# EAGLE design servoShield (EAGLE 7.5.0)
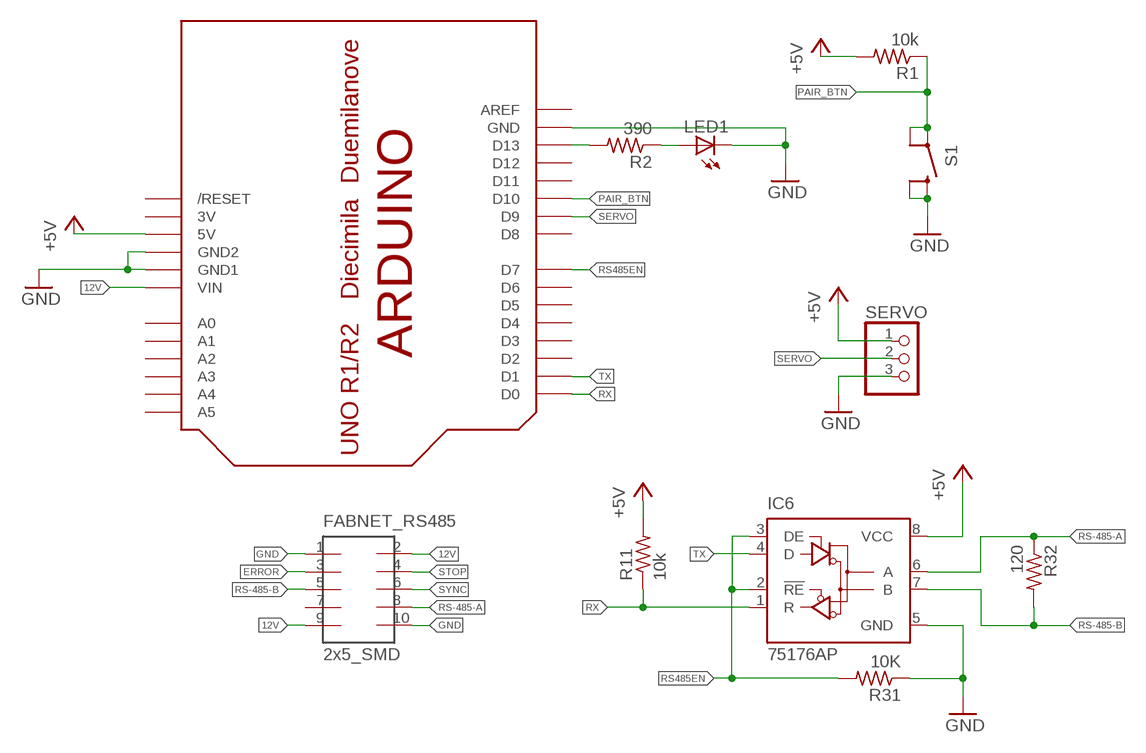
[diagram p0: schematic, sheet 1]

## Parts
FABNET_RS485  2x5_SMD  2X5HEADER  [2X5_SMD]
IC6  75176AP  [DIL08]
LED1  LEDCHIPLED_1206  [CHIPLED_1206]
R1  10k  R-US_R1206  [R1206]
R2  390  R-US_R1206  [R1206]
R11  10k  R-US_R1206  [R1206]
R31  10K  R-US_R1206  [R1206]
R32  120  R-US_R0805  [R0805]
S1  SWITCH-MOMENTARY-2  [TACTILE_SWITCH_TALL]
SERVO  PINHD-1X3  [1X03]
U$1  ARDUINOUNO  [ARDUINO]

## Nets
12V: FABNET_RS485.2 FABNET_RS485.9 U$1.VIN
+5V: IC6.8(VCC) R1.2 R11.2 SERVO.1 U$1.5V
ERROR: FABNET_RS485.3
GND: FABNET_RS485.1 FABNET_RS485.10 IC6.5(GND) LED1.C R31.1 S1.B1 S1.B2 SERVO.3 U$1.GND U$1.GND1 U$1.GND2
N$1: R2.2 U$1.D13
N$2: LED1.A R2.1
PAIR_BTN: R1.1 S1.A1 S1.A2 U$1.D10
RS485EN: IC6.2(!RE) IC6.3(DE) R31.2 U$1.D7
RS-485-A: FABNET_RS485.8 IC6.6(A) R32.1
RS-485-B: FABNET_RS485.5 IC6.7(B) R32.2
RX: IC6.1(R) R11.1 U$1.D0
SERVO: SERVO.2 U$1.D9
STOP: FABNET_RS485.4
SYNC: FABNET_RS485.6
TX: IC6.4(D) U$1.D1
Unconnected: FABNET_RS485.7 U$1.A0 U$1.A1 U$1.A2 U$1.A3 U$1.A4 U$1.A5 U$1.AREF U$1.D2 U$1.D3 U$1.D4 U$1.D5 U$1.D6 U$1.D8 U$1.D11 U$1.D12 U$1.RESET(/RESET)

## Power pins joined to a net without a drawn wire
3V: U$1.3V

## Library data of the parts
FABNET_RS485 = mellis:2X5HEADER
IC6 = 751xx:75176A: DIFFERENTIAL BUS TRANSCEIVER Source: http://focus.ti.com/lit/ds/symlink/sn75176a.pdf
LED1 = led:LED: LED
R1 R2 R11 R31 R32 = rcl:R-US_: RESISTOR, American symbol
S1 = SparkFun-Electromechanical_2:SWITCH-MOMENTARY-2: Various NO switches- pushbuttons, reed, etc
SERVO = pinhead:PINHD-1X3: PIN HEADER
U$1 = adafruit:ARDUINO: Arduino Diecimila/Duemilanove Make a shield with ease, this package has all the named pins as well as the two mounting drill holes and an outline of the USB and DC power connector. The outline is on the DIMENSION layer, so if your board house uses it they will cut the outline to match.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

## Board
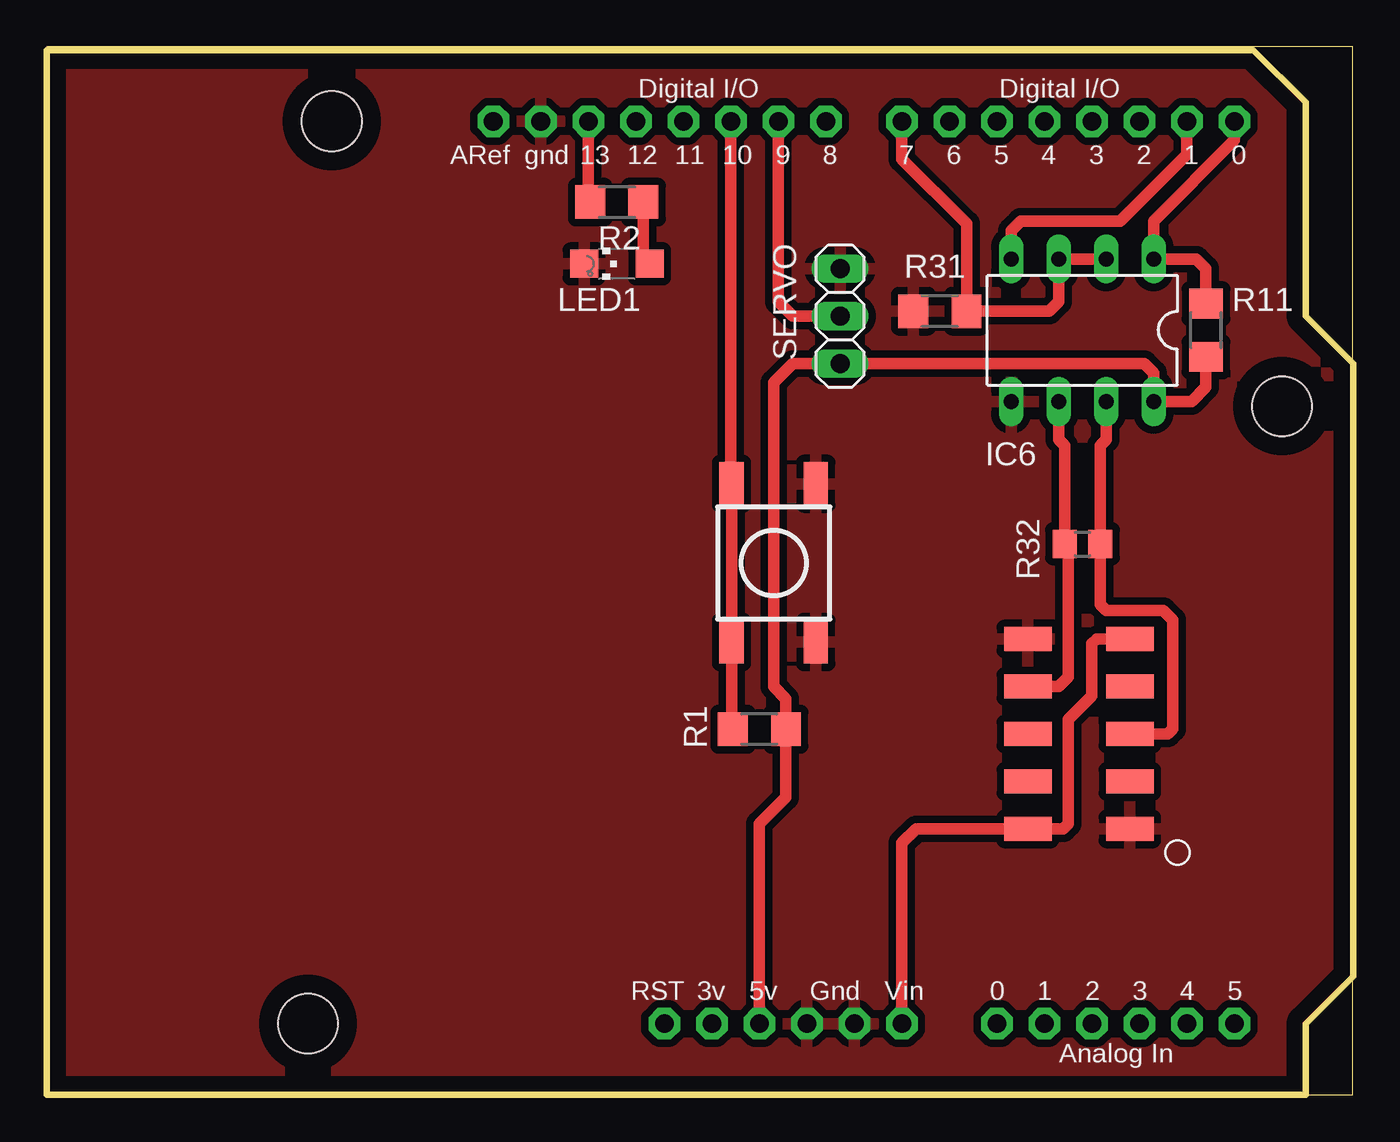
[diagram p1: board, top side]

Size 69.85 x 56.06 mm. Coordinates in mm from the lower left corner, seen from the top.
Outline: 0,0 69.83,0 69.83,56.06 0,56.06 0,0
Copper layers (1*16): Top 0.035mm / dielectric 1.5mm / Bottom 0.035mm
Design rules "default *": minimum track width 10mil, minimum drill 24mil, track to track 16mil, track to pad 16mil, pad to pad 16mil, via to via 16mil, smd to smd 16mil, copper to edge 40mil, drill to drill 8mil, minimum pad ring 10mil, minimum via ring 8mil, stop-mask expansion 4mil, vias tented up to drill 0mil, thermal gap 16mil
Milling: 9 lines

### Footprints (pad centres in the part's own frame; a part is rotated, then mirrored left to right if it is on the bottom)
2X5_SMD = smd 2.54 x 1.27: 1 -2.54,5.08; 2 2.92,5.08; 3 -2.54,2.54; 4 2.92,2.54; 5 -2.54,0; 6 2.92,0; 7 -2.54,-2.54; 8 2.92,-2.54; 9 -2.54,-5.08; 10 2.92,-5.08
DIL08 = drill 0.813 long: 1 -3.81,-3.81; 2 -1.27,-3.81; 3 1.27,-3.81; 4 3.81,-3.81; 5 3.81,3.81; 6 1.27,3.81; 7 -1.27,3.81; 8 -3.81,3.81
CHIPLED_1206 = smd 1.5 x 1.5: A 0,-1.75; C 0,1.75
R1206 = smd 1.6 x 1.803: 1 -1.422,0; 2 1.422,0
R0805 = smd 1.3 x 1.5: 1 -0.95,0; 2 0.95,0
TACTILE_SWITCH_TALL = smd 2.312 x 1.3: A1 -4.229,-2.25; A2 4.229,-2.25; B1 -4.229,2.25; B2 4.229,2.25
1X03 = drill 1.016 long: 1 -2.54,0; 2 0,0; 3 2.54,0
ARDUINO = drill 1 pad 1.676 octagon: 3V 35.56,2.54; 5V 38.1,2.54; A0 50.8,2.54; A1 53.34,2.54; A2 55.88,2.54; A3 58.42,2.54; A4 60.96,2.54; A5 63.5,2.54; AREF 23.876,50.8; D0 63.5,50.8; D1 60.96,50.8; D2 58.42,50.8; D3 55.88,50.8; D4 53.34,50.8; D5 50.8,50.8; D6 48.26,50.8; D7 45.72,50.8; D8 41.656,50.8; D9 39.116,50.8; D10 36.576,50.8; D11 34.036,50.8; D12 31.496,50.8; D13 28.956,50.8; GND 26.416,50.8; GND1 43.18,2.54; GND2 40.64,2.54; RESET 33.02,2.54; VIN 45.72,2.54 | hole 3.2: 15.24,50.8; 66.04,35.56; 13.97,2.54

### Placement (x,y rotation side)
FABNET_RS485  55.37,19.3 180 top
IC6  55.37,40.89 180 top
LED1  30.48,44.45 90 top
R1  38.1,19.56 0 top
R2  30.48,47.75 180 top
R11  61.98,40.89 270 top
R31  47.75,41.91 0 top
R32  55.37,29.46 0 top
S1  38.86,28.45 270 top
SERVO  42.42,41.66 90 top
U$1  0,1.27 0 top

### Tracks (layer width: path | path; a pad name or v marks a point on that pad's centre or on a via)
12V
  Top 0.61: FABNET_RS485.9 56.13,24.38 55.88,24.13 55.88,21.34 54.61,20.07 54.61,14.48 54.36,14.22 FABNET_RS485.2 46.48,14.22 45.72,13.46 U$1.VIN
+5V
  Top 0.61: U$1.5V 38.1,14.48 39.52,15.9 R1.2 39.52,21.18 38.86,21.84 38.86,38.1 39.88,39.12 SERVO.1 58.67,39.12 59.18,38.61 IC6.8 61.21,37.08 61.98,37.85 R11.2
GND
  pour Top: 0,0 67.31,0 67.31,3.81 69.85,6.35 69.85,39.12 67.31,41.66 67.31,53.09 64.52,55.88 0,55.88
N$1
  Top 0.61: U$1.D13 28.96,47.85 R2.2
N$2
  Top 0.61: R2.1 31.9,44.78 LED1.A
PAIR_BTN
  Top 0.61: U$1.D10 36.58,32.71 S1.A1 S1.A2 36.61,19.62 R1.1
RS485EN
  Top 0.61: IC6.2 IC6.3 54.1,42.42 53.59,41.91 R31.2 49.17,46.58 45.72,50.04 U$1.D7
RS-485-A
  Top 0.61: FABNET_RS485.8 54.1,21.84 54.61,22.35 54.61,29.28 R32.1 54.42,34.73 54.1,35.05 IC6.6
RS-485-B
  Top 0.61: FABNET_RS485.5 59.94,19.3 60.2,19.56 60.2,25.4 59.69,25.91 56.64,25.91 56.32,26.23 R32.2 56.32,34.73 56.64,35.05 IC6.7
RX
  Top 0.61: U$1.D0 63.5,51.05 59.18,46.74 IC6.1 61.47,44.7 61.98,44.2 R11.1
SERVO
  Top 0.61: SERVO.2 39.88,41.66 39.12,42.42 U$1.D9
TX
  Top 0.61: IC6.4 51.56,46.23 52.07,46.74 57.4,46.74 60.96,50.29 U$1.D1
